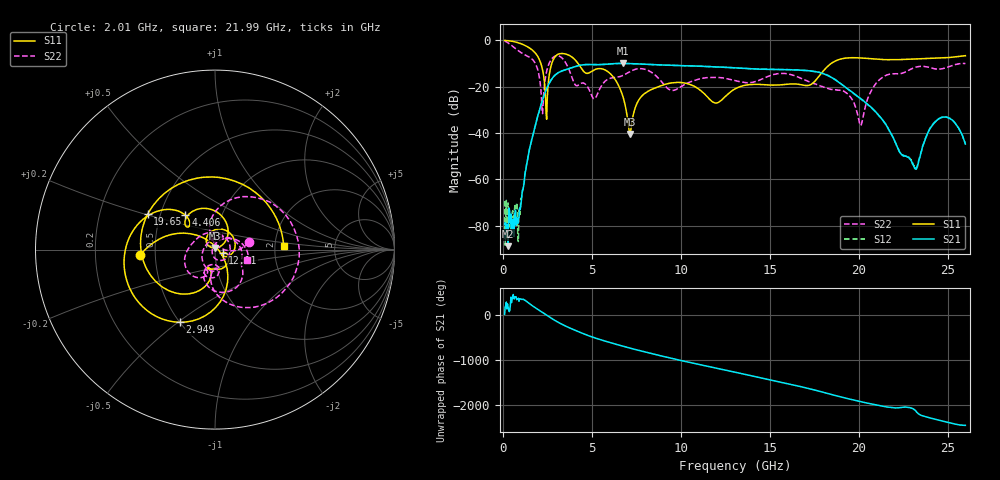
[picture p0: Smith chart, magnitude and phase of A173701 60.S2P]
!  2-Port S-parameters saved by WinCal
! VAR MeasName=S-Parameters (CALIBRATED_DATA) read from VNA (N5245A)
! VAR MeasDate=2017-6-7 10:32:24
! VAR NAME=A173701 60
! VAR FILENAME=A173701 60.S2P
! VAR DATE=2017-6-7 10:32:24
! VAR PHYS_PORTS=1,2
# Hz S DB R 50
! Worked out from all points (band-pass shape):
!   801 points, 100 MHz to 26 GHz, reference 50 ohm
!   highest |S21| = -9.91 dB at 6.769 GHz (marker M1); lowest = -88.9 dB at 294.2 MHz (marker M2)
!   |S21| within 3 dB of the highest: 3.422 GHz to 16.77 GHz (13.35 GHz wide, 132 % of centre); 16.78032 GHz to 16.81773 GHz (37.4 MHz wide, 0.223 % of centre)
!   lowest |S11| = -40.4 dB at 7.125 GHz (marker M3), VSWR 1.02, Z = 50.1 + j0.947 ohm
!   |S11| at or under -10 dB: 2.14 GHz to 2.749 GHz (608.3 MHz wide, 24.9 % of centre); 4.231 GHz to 18.45 GHz (14.22 GHz wide, 125 % of centre)
!   |S22| runs from -36.7 to -0.2 dB; largest |S21 - S12| = 0.0039
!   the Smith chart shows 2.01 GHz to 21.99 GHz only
!   S11 on the Smith chart (normalised r, x): 2.01 GHz: 0.41, -0.03; 2.949 GHz: 0.50, -0.51; 4.406 GHz: 0.67, +0.27; 12.11 GHz: 1.09, -0.04; 19.65 GHz: 0.43, +0.20; 21.99 GHz: 2.24, +0.11
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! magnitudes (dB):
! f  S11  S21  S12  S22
! 100 MHz  0.0  -79.6  -69.3  -0.2
! 294.2 MHz  -0.1  -88.9  -70.2  -1.1
! 941.8 MHz  -1.2  -72.5  -75.4  -4.8
! 2.01 GHz  -7.6  -31.4  -31.4  -14.1
! 2.237 GHz  -12.8  -25.6  -25.6  -31.6
! 2.463 GHz  -34.0  -20.9  -20.9  -13.3
! 2.949 GHz  -6.9  -14.9  -14.9  -6.7
! 4.406 GHz  -12.0  -10.6  -10.6  -18.5
! 4.438 GHz  -12.3  -10.6  -10.6  -18.4
! 6.769 GHz  -24.7  -9.9  -9.9  -15.0
! 7.125 GHz  -40.4  -10.0  -10.0  -13.6
! 8.744 GHz  -20.0  -10.6  -10.6  -16.3
! 12.11 GHz  -26.8  -11.5  -11.5  -16.0
! 13.05 GHz  -20.9  -11.9  -11.8  -17.4
! 17.39 GHz  -18.7  -13.3  -13.2  -18.4
! 19.65 GHz  -7.5  -22.5  -22.6  -25.7
! 20.14 GHz  -7.6  -25.3  -25.5  -36.5
! 21.69 GHz  -8.3  -38.4  -38.6  -14.7
! 21.99 GHz  -8.3  -42.8  -42.8  -14.4
! 23.18 GHz  -8.0  -55.1  -55.5  -11.6
! 24.54 GHz  -7.6  -33.8  -33.6  -12.4
! 26 GHz  -6.6  -44.8  -44.6  -10.0
